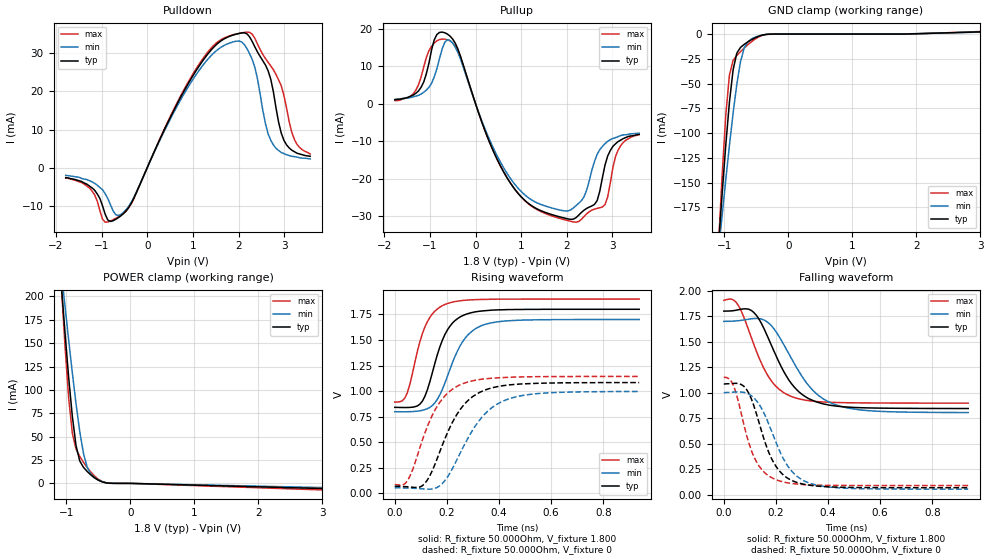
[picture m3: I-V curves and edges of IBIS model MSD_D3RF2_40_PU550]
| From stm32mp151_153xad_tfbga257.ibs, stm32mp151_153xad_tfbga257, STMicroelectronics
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[Model] MSD_D3RF2_40_PU550
Model_type   I/O
C_comp 2.403pF   2.321pF   2.525pF
Vinh = 1.150V
Vinl = 650.000mV
Vmeas = 900.000mV
Vref = 900.000mV
[Model Spec]
Vinh   1.150V   1.100V   1.200V
Vinl   650.000mV   600.000mV   700.000mV
Vmeas   900.000mV   850.000mV   950.000mV
Vref   900.000mV   850.000mV   950.000mV
[Temperature Range]   25.000   125.000   -40.000
[Voltage Range]   1.800V   1.700V   1.900V
[GND Clamp Reference]   0.00V   0.00V   0.00V
[Pulldown Reference]   0.00V   0.00V   0.00V
[POWER Clamp Reference]   1.800V   1.700V   1.900V
[Pullup Reference]   1.800V   1.700V   1.900V
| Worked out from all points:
|   slope of the pulldown table from 0 to 0.27 V, typ, clamps not added: 37.2 ohm
|   slope of the pullup table from 0 to 0.27 V, typ, clamps not added: 29.4 ohm
|   GND clamp passes 1 mA (typ) near -0.40 V on its own axis
|   POWER clamp passes 1 mA (typ) near -0.41 V on its own axis
|   rising waveform, R_fixture 50.000Ohm, V_fixture 1.800: 20-80 % time 77.1ps typ, 95.1ps min, 69.2ps max; typ from 0.841 V to 1.8 V
|   rising waveform, R_fixture 50.000Ohm, V_fixture 0: 20-80 % time 118ps typ, 137ps min, 108ps max; typ from 0.068 V to 1.08 V
|   falling waveform, R_fixture 50.000Ohm, V_fixture 1.800: 20-80 % time 120ps typ, 139ps min, 105ps max; typ from 1.8 V to 0.844 V
|   falling waveform, R_fixture 50.000Ohm, V_fixture 0: 20-80 % time 87.9ps typ, 105ps min, 77.1ps max; typ from 1.08 V to 0.068 V
[GND Clamp]
-1.785V   -902.5mA   -689.8mA   -1.211A
-1.094V   -215.3mA   -221.3mA   -216.1mA
-1.036V   -162.4mA   -184mA     -144mA
-978.8mV  -112.7mA   -147.7mA   -82.66mA
-921.2mV  -68.92mA   -112.7mA   -41.51mA
-863.6mV  -36.11mA   -79.92mA   -26.65mA
-806.1mV  -19.32mA   -50.89mA   -21.68mA
-748.5mV  -13.5mA    -28.03mA   -17.81mA
-690.9mV  -10.44mA   -13.99mA   -14.19mA
-575.8mV  -5.673mA   -4.859mA   -7.667mA
-287.9mV  -73.99uA   -123uA     -58.99uA
3.57V     3.293mA    2.836mA    3.934mA
[Power Clamp]
-1.77V    883.9mA    691mA      1.161A
-1.079V   213mA      227mA      212.9mA
-1.021V   161.5mA    189.8mA    147.4mA
-963.6mV  113.4mA    153.4mA    91.56mA
-906.1mV  71.61mA    118.2mA    53.48mA
-848.5mV  40.42mA    85.13mA    36.67mA
-790.9mV  24.13mA    55.72mA    28.91mA
-733.3mV  17.27mA    32.47mA    22.68mA
-618.2mV  9.14mA     9.901mA    12.17mA
-503mV    3.513mA    3.609mA    4.571mA
-330.3mV  167.9uA    348uA      196.2uA
3.585V    -6.609mA   -5.357mA   -8.396mA
[Pulldown]
-1.785V   -2.6mA     -2mA       -2.7mA
-1.267V   -4.8mA     -3.4mA     -5.3mA
-921.2mV  -12.19mA   -6.8mA     -14.29mA
-575.8mV  -12.6mA    -12.25mA   -12.47mA
1.152V    26.93mA    25.78mA    27.42mA
2.073V    35.36mA    32.95mA    35.37mA
2.361V    31.62mA    26.21mA    33.86mA
2.591V    26.91mA    11.5mA     28.61mA
2.764V    19.9mA     6mA        25.71mA
2.994V    7.2mA      3.7mA      19mA
3.224V    4.2mA      2.9mA      7.4mA
3.57V     3mA        2.3mA      3.6mA
[Pullup]
-1.77V    1.1mA      1.1mA      873.7uA
-1.309V   2.8mA      2.047mA    3.616mA
-1.021V   10.9mA     4.389mA    14.22mA
-848.5mV  18.49mA    9.339mA    16.83mA
-618.2mV  18.64mA    17.11mA    17.12mA
-387.9mV  14.67mA    13.71mA    14.13mA
763.6mV   -21.21mA   -19.96mA   -21.18mA
2.145V    -30.84mA   -27.84mA   -31.6mA
2.606V    -26.91mA   -15.39mA   -28.18mA
2.779V    -19.8mA    -11.41mA   -27.6mA
3.124V    -10.1mA    -8.779mA   -12.36mA
3.585V    -8.2mA     -7.9mA     -8.247mA
[Ramp]
R_load=50.000Ohm
dV/dt_r   591.600mV/98.500ps  552.243mV/117.000ps  617.334mV/89.000ps
dV/dt_f   591.600mV/104.500ps  552.210mV/123.000ps  617.334mV/91.000ps
[Rising waveform]
R_fixture=50.000Ohm
V_fixture=1.800
V_fixture_min=1.700
V_fixture_max=1.900
0s        841mV      798.5mV    892.5mV
29ps      839.4mV    797.6mV    905mV
48ps      839.3mV    797.9mV    982.8mV
106ps     901.6mV    812.1mV    1.562V
125ps     1.011V     827.5mV    1.678V
154ps     1.272V     885.4mV    1.782V
192ps     1.551V     1.076V     1.847V
259ps     1.736V     1.478V     1.886V
345ps     1.786V     1.651V     1.897V
938ps     1.8V       1.7V       1.9V
[Rising waveform]
R_fixture=50.000Ohm
V_fixture=0
0s        68.02mV    53.44mV    85.7mV
48ps      64.17mV    51.83mV    120.5mV
115ps     95.85mV    42.3mV     585.7mV
144ps     221.9mV    42.49mV    764mV
183ps     474.6mV    97.18mV    924.3mV
250ps     816.1mV    388.3mV    1.061V
345ps     1.009V     774.5mV    1.119V
441ps     1.061V     926.6mV    1.135V
585ps     1.078V     982.2mV    1.142V
938ps     1.083V     996.2mV    1.143V
[Falling waveform]
R_fixture=50.000Ohm
V_fixture=1.800
V_fixture_min=1.700
V_fixture_max=1.900
0s        1.799V     1.698V     1.905V
48ps      1.808V     1.703V     1.883V
68ps      1.818V     1.709V     1.794V
115ps     1.786V     1.726V     1.474V
183ps     1.462V     1.655V     1.114V
259ps     1.09V      1.337V     962.2mV
345ps     919.1mV    1.014V     915mV
441ps     865.1mV    870.8mV    902.3mV
595ps     847.9mV    816.6mV    897.9mV
938ps     843.8mV    804mV      896.5mV
[Falling waveform]
R_fixture=50.000Ohm
V_fixture=0
0s        1.084V     999.3mV    1.149V
39ps      1.09V      1.005V     1.058V
87ps      1.032V     994.7mV    586.2mV
106ps     936.7mV    969.4mV    430.9mV
135ps     708mV      887.1mV    281mV
163ps     478.2mV    750mV      201mV
192ps     310.2mV    565.9mV    155mV
259ps     140.6mV    234.5mV    109.5mV
345ps     86.58mV    99.81mV    93.56mV
938ps     67.52mV    53.06mV    88.62mV
